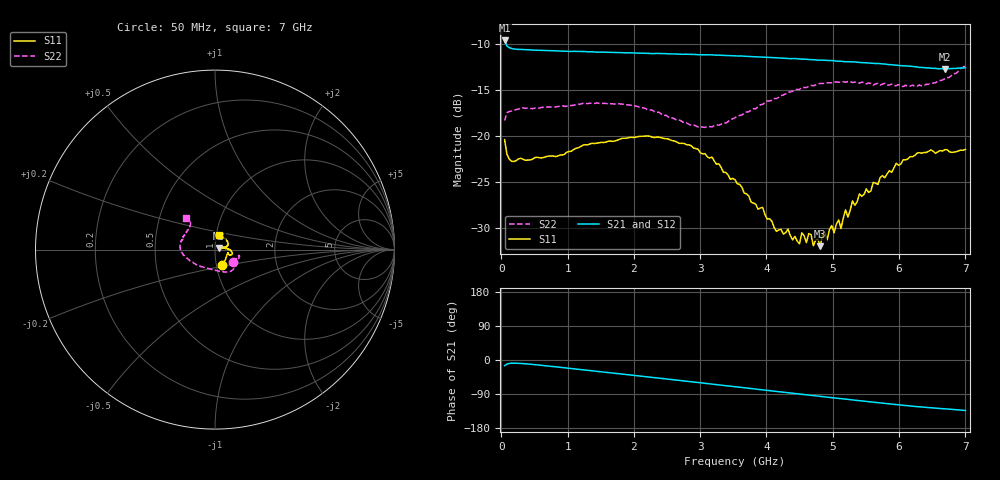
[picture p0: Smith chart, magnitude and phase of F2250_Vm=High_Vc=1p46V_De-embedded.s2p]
! Integrated Device Technology
! Corporate Headquarters
! 6024 Silver Creek Valley Road
! San Jose, CA 95138  USA
! Phone:  1-408-284-8200
! Toll Free:  1-800-223-1366
! Webpage:  http://www.idt.com/
! Timing and RF Division
! 515 Groton Road, Suite 102
! Westford, MA 01886-6024
! Device:  F2250
! Description: Voltage Variable RF Attenuator
! Frequency:  50.0 -  6000.00 MHz
! Package:  3x3 mm Thin QFN Plastic Package: 16 pin
! Ports:  2 RF, 3 DC
!  Pin  1  = GND
!  Pin  2  = NC
!  Pin  3  = RF1  = Port 1
!  Pin  4  = NC
!  Pin  5  = GND
!  Pin  6  = GND
!  Pin  7  = GND
!  Pin  8  = GND
!  Pin  9  = NC
!  Pin 10  = RF2  = Port 2
!  Pin 11  = NC
!  Pin 12  = GND
!  Pin 13  = GND
!  Pin 14  = VCNTRL
!  Pin 15  = VDD
!  Pin 16  = VMODE
! Vcntrl:  1.460 Volts
! Vmode:  +3.300 Volts
! Vdd:  +3.30  Volts
! Current:  1.329 mA
! Data:  The device was measured on a the F2250 evaluation board which has
!  individual transmission lines to the RF pins.  Data was collected
!  using a calibrated network analyzer.  The evaluation board was
!  de-embedded using a TRL calibration technique.
!  The reference plane is the edge of the package pin.
! Misc:  SN 10
!  Action Tracker AT0258
! Date Measured:  2014-11-26
! Date:  2015-10-15  MJV
! Note:
!  Integrated Device Technology supplies this data as a sample of measured
!  data at the package pin for this product.  Your particular data for this
!  product may vary.
!  Data was taken at 25 degrees C.
!  Integrated Device Technology reserves the right to change this data at anytime.
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# GHz S dB R 50
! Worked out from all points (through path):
!   201 points, 50 MHz to 7 GHz, reference 50 ohm
!   highest |S21| = -9.62 dB at 50 MHz (marker M1); lowest = -12.7 dB at 6.687 GHz (marker M2)
!   group delay of S21, straight-line fit = 53 ps
!   lowest |S11| = -32.0 dB at 4.811 GHz (marker M3), VSWR 1.05, Z = 52.4 + j0.969 ohm
!   |S11| at or under -10 dB: start of sweep to end of sweep
!   |S22| runs from -19.1 to -12.3 dB; largest |S21 - S12| = 0.0013
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0.05  -20.42 -67.2  -9.62 -15.0  -9.63 -15.0  -18.36 -35.1
0.08475  -21.99 -41.8  -10.22 -10.8  -10.24 -10.8  -17.49 -19.5
0.189  -22.81 -21.7  -10.54 -8.4  -10.54 -8.4  -17.22 -13.5
1.2315  -21.03 -19.8  -10.82 -25.8  -10.83 -25.8  -16.47 -41.9
2.37825  -20.17 -10.8  -11.04 -47.8  -11.05 -47.8  -17.44 -69.2
2.969  -21.48 -0.6  -11.17 -59.5  -11.16 -59.5  -19.05 -97.2
3.525  -24.79 8.6  -11.31 -70.6  -11.30 -70.6  -18.04 -132.9
4.1505  -30.42 22.4  -11.51 -82.9  -11.51 -83.0  -15.94 -161.0
4.32425  -30.17 24.0  -11.59 -86.3  -11.59 -86.4  -15.25 -166.7
4.498  -31.77 22.3  -11.64 -89.8  -11.63 -89.8  -14.95 -171.8
4.53275  -30.58 22.7  -11.66 -90.5  -11.62 -90.6  -14.76 -172.7
4.60225  -31.64 24.9  -11.67 -91.9  -11.68 -91.9  -14.76 -174.3
4.67175  -30.76 31.2  -11.71 -93.2  -11.72 -93.2  -14.52 -175.7
4.7065  -31.99 28.7  -11.71 -93.9  -11.73 -93.9  -14.55 -176.4
4.81075  -32.03 21.7  -11.76 -95.9  -11.74 -95.9  -14.30 -178.4
4.8455  -30.73 16.6  -11.77 -96.6  -11.75 -96.6  -14.30 -179.2
4.9845  -29.79 21.7  -11.81 -99.4  -11.83 -99.4  -14.24 176.7
5.1235  -30.12 17.1  -11.88 -102.0  -11.89 -102.0  -14.13 173.8
5.29725  -27.11 12.6  -11.95 -105.3  -11.96 -105.4  -14.20 170.2
5.85325  -23.81 13.6  -12.25 -115.7  -12.25 -115.9  -14.47 155.0
6.68725  -21.52 44.9  -12.73 -128.8  -12.72 -128.9  -13.79 132.1
7  -21.49 75.9  -12.60 -133.2  -12.59 -133.4  -12.34 132.3
